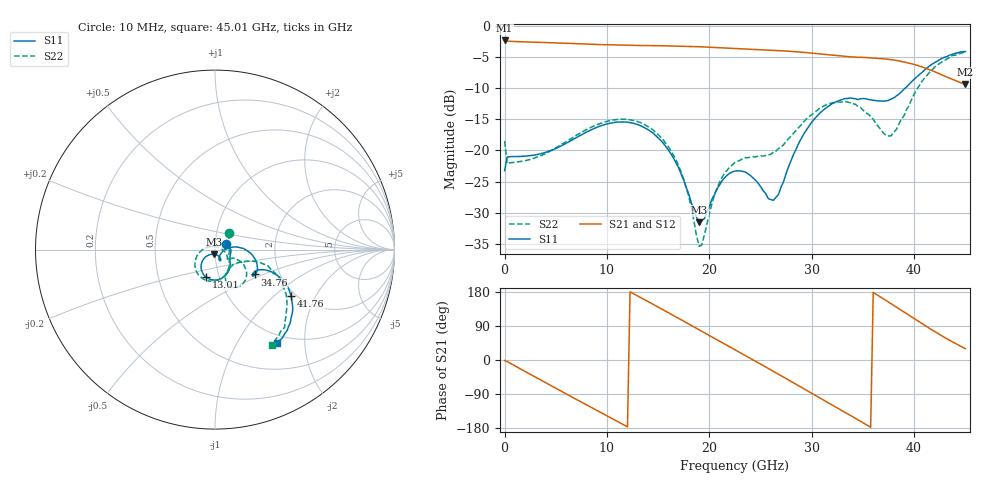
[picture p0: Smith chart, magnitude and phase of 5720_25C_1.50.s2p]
! Device:  ADRF5720
! Description: 0.5dB LSB GaAs MMIC 6-bit Digital Attenuator
! Frequency:  0.000009 -  40 GHz
! Ports:
!	RF1	= Port 1
!	RF2	= Port 2
! Vdd:  3.3 Volt
! Vss:  -3.3 Volt
! Control:  0/3.3 Volt
! State:  1.50 dB attenuation
! Data:  The device was measured using G-S-G Probes on a matrix board.
!  Data was collected using an calibrated 4 port network analyzer.
!  The reference plane for this measurement is at the launchers.
! Note:  Analog Devices supplies this data as a sample of measured data
!  for this product.  Your particular data for this product may vary.
!  Data was taken at 25 degrees C.
!  Analog Devices reserves the right to change this data at anytime.
# GHZ S DB R 45.0
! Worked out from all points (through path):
!   181 points, 10 MHz to 45.01 GHz, reference 45 ohm
!   highest |S21| = -2.31 dB at 10 MHz (marker M1); lowest = -9.4 dB at 45.01 GHz (marker M2)
!   group delay of S21, straight-line fit = 42.5 ps
!   lowest |S11| = -31.6 dB at 19.01 GHz (marker M3), VSWR 1.05, Z = 44.4 - j2.27 ohm
!   |S11| at or under -10 dB: start of sweep to 39.12 GHz
!   |S22| runs from -35.4 to -4.2 dB; largest |S21 - S12| = 0.00093
!   S11 on the Smith chart (normalised r, x): 10 MHz: 1.13, +0.07; 13.01 GHz: 0.87, -0.27; 34.76 GHz: 1.49, -0.44; 41.76 GHz: 1.90, -1.28; 45.01 GHz: 0.87, -1.48
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0.01  -23.25 26.9  -2.31 -1.3  -2.31 -1.3  -18.51 50.4
0.26  -21.07 -0.3  -2.43 -4.2  -2.43 -4.2  -22.11 -0.1
2.01  -20.92 -17.2  -2.54 -30.3  -2.54 -30.3  -21.65 -17.8
4.26  -20.17 -32.0  -2.66 -63.5  -2.66 -63.5  -20.28 -34.8
6.01  -18.85 -42.1  -2.76 -89.2  -2.76 -89.2  -18.60 -47.4
7.76  -17.25 -54.8  -2.87 -114.8  -2.87 -114.8  -16.85 -62.3
10.51  -15.56 -80.8  -3.03 -154.7  -3.03 -154.7  -15.14 -90.6
13.01  -15.84 -107.6  -3.12 169.0  -3.12 169.0  -15.36 -120.3
15.26  -18.39 -130.1  -3.16 135.9  -3.16 135.9  -17.87 -149.7
17.26  -23.83 -142.3  -3.23 106.0  -3.23 106.0  -23.52 178.7
19.01  -31.58 -104.5  -3.32 79.7  -3.32 79.7  -35.40 96.3
21.01  -25.53 -57.6  -3.47 49.6  -3.47 49.6  -25.06 -12.0
22.76  -23.28 -64.1  -3.61 23.2  -3.61 23.3  -21.73 -32.3
26.26  -28.03 -30.2  -3.89 -29.9  -3.89 -29.9  -20.27 -31.0
28.26  -20.52 8.1  -4.10 -60.8  -4.10 -60.8  -17.17 -24.2
30.26  -14.95 -1.6  -4.39 -91.9  -4.39 -91.9  -13.87 -32.2
32.26  -12.26 -17.7  -4.71 -122.7  -4.72 -122.7  -12.30 -48.2
34.76  -11.69 -32.1  -5.01 -161.4  -5.01 -161.3  -13.08 -67.9
37.76  -11.73 -27.3  -5.40 148.6  -5.40 148.7  -17.65 -40.0
39.76  -8.94 -22.2  -6.06 113.7  -6.06 113.7  -11.78 -16.0
41.76  -6.12 -31.2  -7.17 79.2  -7.17 79.3  -7.04 -29.8
45.01  -4.09 -56.7  -9.37 29.8  -9.37 29.9  -4.17 -59.1
